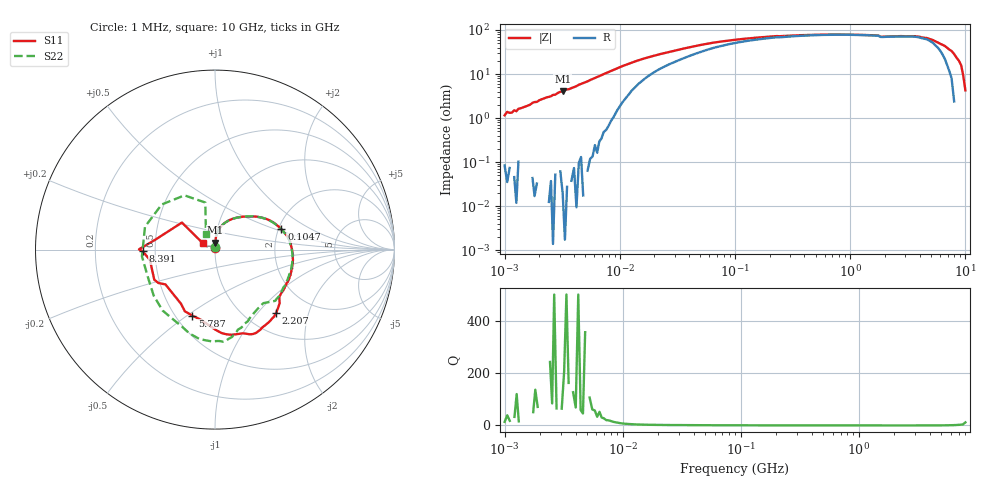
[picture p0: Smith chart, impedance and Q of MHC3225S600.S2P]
!Agilent Technologies,E5071C,MY46111244,A.11.31
!Date: Thu May 09 18:30:44 2019
!Data & Calibration Information:
!Freq	S11:SOLT2(ON)	S21:SOLT2(ON)	S12:SOLT2(ON)	S22:SOLT2(ON)
# Hz S dB R 50
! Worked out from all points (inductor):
!   201 points, 1 MHz to 10 GHz, reference 50 ohm
!   read as one part in series: L = 192 nH near 1.053 MHz
!   highest Q = 163 at 3.193 MHz (marker M1), where L = 202 nH
!   S11 on the Smith chart (normalised r, x): 1 MHz: 1.00, +0.02; 104.7 MHz: 2.08, +0.56; 2.207 GHz: 1.36, -1.26; 5.787 GHz: 0.61, -0.52; 8.391 GHz: 0.43, -0.01; 10 GHz: 0.87, +0.06
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1000000  -38.77 85.2  0.00 -0.7  -0.02 -0.6  -38.62 87.1
1053043  -37.38 89.6  -0.03 -0.8  0.02 -0.9  -38.36 87.1
1106086  -38.15 86.1  -0.01 -0.8  -0.01 -0.8  -37.87 90.3
1159128  -37.29 91.3  0.01 -0.8  -0.02 -0.6  -36.66 92.3
3192505  -28.07 87.4  -0.01 -2.3  -0.00 -2.4  -27.97 86.6
4810209  -24.25 85.8  -0.02 -3.7  -0.02 -3.6  -24.25 86.4
1.053043e7  -16.76 73.0  -0.29 -8.4  -0.29 -8.4  -16.80 73.0
2.206931e7  -12.38 49.7  -1.26 -12.7  -1.26 -12.7  -12.39 49.7
1.047129e8  -8.24 17.1  -3.80 -13.1  -3.80 -13.1  -8.24 16.9
4.810209e8  -7.23 -4.4  -4.97 -11.6  -4.99 -11.6  -7.26 -5.2
1.44544e9  -7.07 -29.0  -5.18 -22.3  -5.19 -22.4  -7.15 -32.3
2.206931e9  -6.20 -45.8  -5.37 -33.6  -5.38 -33.6  -7.74 -56.2
3.801894e9  -5.85 -67.7  -6.09 -50.4  -6.11 -50.4  -6.26 -77.7
4.83488e9  -6.63 -85.6  -6.06 -63.1  -6.08 -63.0  -5.86 -87.4
5.786901e9  -8.20 -108.8  -5.59 -77.9  -5.60 -78.0  -5.93 -99.9
6.952868e9  -9.44 -144.9  -4.94 -98.5  -4.88 -98.7  -6.98 -130.8
7.585776e9  -8.46 -153.6  -4.36 -109.2  -4.35 -109.1  -7.84 -156.0
8.390517e9  -7.91 -178.7  -3.81 -124.5  -3.82 -124.5  -7.74 161.9
8.792888e9  -7.46 179.8  -3.08 -132.8  -3.06 -132.8  -8.20 139.7
9.195259e9  -9.57 169.8  -2.26 -143.3  -2.33 -143.4  -9.20 119.4
9.597629e9  -12.47 140.7  -1.61 -156.5  -1.62 -156.6  -11.45 101.6
1e10  -22.20 152.1  -1.05 -172.5  -1.05 -172.4  -19.91 119.9
